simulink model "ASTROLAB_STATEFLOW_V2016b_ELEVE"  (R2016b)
settings: Solver=VariableStepAuto  StartTime=0.0  StopTime=inf  FixedStep=1e-3  MaxStep=0.001  RelTol=1e-3  EnableMultiTasking=on
undefined symbols (not defined in the file): ASTROLAB, CARTER, deg, EMBASE, f, fourche, kg, m, N, r, rad, RootGround, RootPart, s, SIM, STL, tube
libraries: mblibv1 x14, powerlib_meascontrol x4, simulink_extras x4, simulink x1

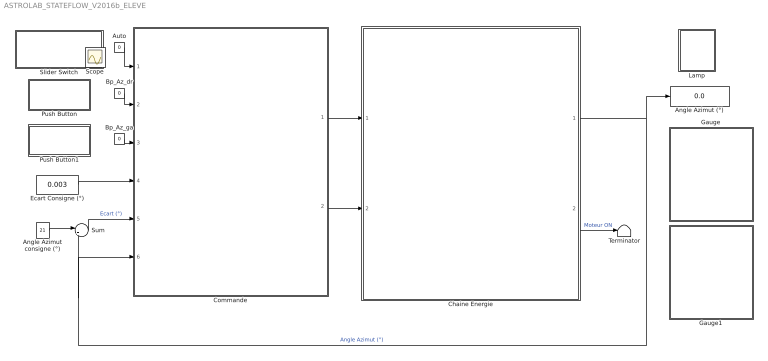
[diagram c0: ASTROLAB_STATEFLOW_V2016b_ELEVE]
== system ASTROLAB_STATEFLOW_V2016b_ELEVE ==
  Angle Azimut consigne (°) : Constant  Value=21
  Angle Azimut (°) : Display
  Auto : Constant  Value=0
  Bp_Az_dr : Constant  Value=0
  Bp_Az_ga : Constant  Value=0
  Chaine Energie : Subsystem
  Commande : Stateflow chart  TreatAsAtomicUnit=on
  Ecart Consigne (°) : Constant  Value=0.003
  Gauge : Subsystem  DialogController=hmiCreateDDGDialog  IsWebBlock=on
  Gauge1 : Subsystem  DialogController=hmiCreateDDGDialog  IsWebBlock=on
  Lamp : Subsystem  DialogController=hmiCreateDDGDialog  IsWebBlock=on
  Push Button : Subsystem  DialogController=hmiCreateDDGDialog  IsWebBlock=on
  Push Button1 : Subsystem  DialogController=hmiCreateDDGDialog  IsWebBlock=on
  Slider Switch : Subsystem  DialogController=hmiCreateDDGDialog  IsWebBlock=on
  Sum : Sum  Inputs=|+-
  Terminator : Terminator
  Scope : Scope
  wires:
  Commande/1(vitesse_azimut) -> Chaine Energie/1(vitesse_azimut)
  Commande/2(sens_azimut) -> Chaine Energie/2(sens_azimut)
  Chaine Energie/1(position_azimut) -> Commande/6(angle_az), Sum/2, Angle Azimut (°)/1  "Angle Azimut (°)"
  Angle Azimut consigne (°)/1 -> Sum/1
  Sum/1 -> Commande/5(e_az)  "Ecart (°)"
  Ecart Consigne (°)/1 -> Commande/4(e_az_cons)
  Auto/1 -> Commande/1(auto)
  Bp_Az_dr/1 -> Commande/2(bp_az_droite)
  Bp_Az_ga/1 -> Commande/3(bp_az_gauche)
  Chaine Energie/2(moteur_on) -> Terminator/1  "Moteur ON"

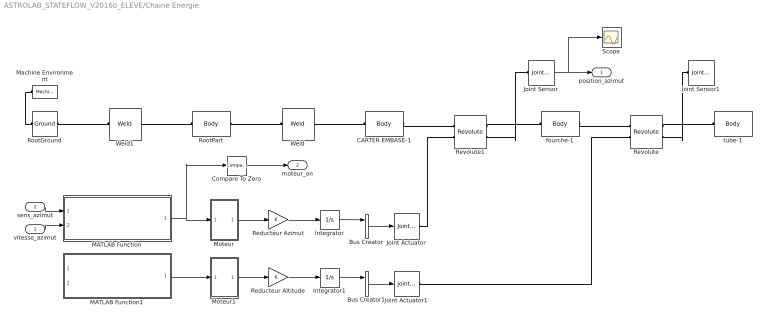
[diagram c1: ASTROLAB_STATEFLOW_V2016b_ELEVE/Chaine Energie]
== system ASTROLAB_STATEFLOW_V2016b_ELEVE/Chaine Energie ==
  vitesse_azimut : Inport
  sens_azimut : Inport  Port=2
  Bus Creator : BusCreator  Inputs=3
  Bus Creator1 : BusCreator  Inputs=3
  CARTER EMBASE-1 : mblibv1/Bodies/Body  LConnTagsString=CS2  RConnTagsString=CS3  UpdateFromCAD=on  PMImportedID=CARTER EMBASE-1  DialogClass=MechanicalBodyBlock  Mass=0.499764  MassUnits=kg  InertiaUnits=kg*m^2  Inertia=[0.0012574,-3.27626e-05,-2.02056e-06;-3.27626e-05,0.00181958,9.31617e-06;-2.02056e-06,9.31617e-06,0.00114593]  Shape=Cylinder  ShapeDims=[1 1]  ShapeUnits=m  ShapeUse=false  Density=1  DensityUnits=kg/m^3  DensityUse=false  GraphicsMode=GFXFILE  GraphicsFileName=STL/ASTROLAB-SIM - CARTER EMBASE-1.STL  BodyColorSelMode=COLORPALETTE  BodyColor=[0.313725;0.313725;0.313725]  AttachedToCS=CS1  CG=Right$CG$[0.000443056 -0.0440147 0.00175883]$WORLD$WORLD$m$[-1 0 0;0 1 0;0 0 -1]$3x3 Transform$rad$WORLD$false$CARTER EMBASE-1::CG(AUTOGEN)  WorkingFrames=Right$CS1$[-0.0385593 -0.0337526 0]$WORLD$WORLD$m$[-1 0 0;0 1 0;0 0 -1]$3x3 Transform$rad$WORLD$false$CARTER EMBASE-1::CS1(AUTOGEN)#Left$CS2$[0.000443056 -0.0440147 0.00175883]$WORLD$WORLD$m$[1 0 0;0 1 0;0 0 1]$3x3 Transform$rad$WORLD$true$ASTROLAB-SIM/RootPart:-:CARTER EMBASE-1::CARTER EMBASE-1(AUTOGEN)#Right$CS3$[0 -0.009 0]$WORLD$WORLD$m$[1 0 0;0 1 0;0 0 1]$3x3 Transform$rad$WORLD$true$CARTER E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  CGPos=[0.000443056 -0.0440147 0.00175883]  CGRot=[-1 0 0;0 1 0;0 0 -1]  CS0Pos=[]  CS0Rot=[]  CS1Pos=[-0.0385593 -0.0337526 0]  CS1Rot=[-1 0 0;0 1 0;0 0 -1]  CS2Pos=[0.000443056 -0.0440147 0.00175883]  CS2Rot=[1 0 0;0 1 0;0 0 1]  CS3Pos=[0 -0.009 0]  CS3Rot=[1 0 0;0 1 0;0 0 1]  CS4Pos=[]  CS4Rot=[]  CS5Pos=[]  CS5Rot=[]  CS6Pos=[]  CS6Rot=[]  CS7Pos=[]  CS7Rot=[]  CS8Pos=[]  CS8Rot=[]  CS9Pos=[]  CS9Rot=[]  CS10Pos=[]  CS10Rot=[]  CS11Pos=[]  CS11Rot=[]  CS12Pos=[]  CS12Rot=[]  CS13Pos=[]  CS13Rot=[]  CS14Pos=[]  CS14Rot=[]  CS15Pos=[]  CS15Rot=[]  CS16Pos=[]  CS16Rot=[]  CS17Pos=[]  CS17Rot=[]  CS18Pos=[]  CS18Rot=[]  CS19Pos=[]  CS19Rot=[]  CS20Pos=[]  CS20Rot=[]
  Compare To Zero : simulink/Logic and Bit Operations/Compare To Zero  relop===  OutDataTypeStr=boolean
  Integrator : Integrator
  Integrator1 : Integrator
  Joint Actuator : mblibv1/Sensors &  Actuators/Joint Actuator  UpdateFromCAD=off  PhysicalDomain=Mechanical  PortType=blob  ActuationStyle=Motion  AngleUnits=rad  ArcVelocityUnits=rad/s  ArcAccelerationUnits=rad/s^2  CoordPositionUnits=m  VelocityUnits=m/s  AccelerationUnits=m/s^2  ForceUnits=N  TorqueUnits=N*m  ActiveIO=on  Width=3  DialogClass=MechanicalActuatorBlock  Primitive=R1  ReferenceFrame=Absolute (World)
  Joint Actuator1 : mblibv1/Sensors &  Actuators/Joint Actuator  UpdateFromCAD=off  PhysicalDomain=Mechanical  PortType=blob  ActuationStyle=Motion  AngleUnits=rad  ArcVelocityUnits=rad/s  ArcAccelerationUnits=rad/s^2  CoordPositionUnits=m  VelocityUnits=m/s  AccelerationUnits=m/s^2  ForceUnits=N  TorqueUnits=N*m  ActiveIO=on  Width=3  DialogClass=MechanicalActuatorBlock  Primitive=R1  ReferenceFrame=Absolute (World)
  Joint Sensor : mblibv1/Sensors &  Actuators/Joint Sensor  UpdateFromCAD=off  PhysicalDomain=Mechanical  PortType=blob  Muxed=off  Pose=off  Angle=on  AngleUnits=deg  ArcVelocity=off  ArcVelocityUnits=deg/s  ArcAcceleration=off  ArcAccelerationUnits=deg/s^2  CoordPosition=on  CoordPositionUnits=mm  Velocity=off  VelocityUnits=m/s  Acceleration=off  AccelerationUnits=m/s^2  Quaternion=on  QuaternionDT=off  QuaternionDDT=off  QuaternionUnits=off  OutputVector=[1]  ActiveIO=on  Width=1  DialogClass=MechanicalSensorBlock  Primitive=R1  Force=off  ForceUnits=N  Torque=off  TorqueUnits=N*m  ReferenceFrame=Absolute (World)  ReactionSensedSide=Base  ReactionReferenceFrame=Absolute (World)  ReactionForce=off  ReactionForceUnits=N  ReactionMoment=off  ReactionMomentUnits=N*m
  Joint Sensor1 : mblibv1/Sensors &  Actuators/Joint Sensor  UpdateFromCAD=off  PhysicalDomain=Mechanical  PortType=blob  Muxed=off  Pose=off  Angle=on  AngleUnits=deg  ArcVelocity=off  ArcVelocityUnits=deg/s  ArcAcceleration=off  ArcAccelerationUnits=deg/s^2  CoordPosition=on  CoordPositionUnits=mm  Velocity=off  VelocityUnits=m/s  Acceleration=off  AccelerationUnits=m/s^2  Quaternion=on  QuaternionDT=off  QuaternionDDT=off  QuaternionUnits=off  OutputVector=[1]  ActiveIO=on  Width=1  DialogClass=MechanicalSensorBlock  Primitive=R1  Force=off  ForceUnits=N  Torque=off  TorqueUnits=N*m  ReferenceFrame=Absolute (World)  ReactionSensedSide=Base  ReactionReferenceFrame=Absolute (World)  ReactionForce=off  ReactionForceUnits=N  ReactionMoment=off  ReactionMomentUnits=N*m
  MATLAB Function : MATLAB Function  TreatAsAtomicUnit=on
  MATLAB Function1 : MATLAB Function  TreatAsAtomicUnit=on
  Machine Environment : mblibv1/Bodies/Machine Environment  PortType=env  PhysicalDomain=Mechanical  DialogTemplateClass=MECH.MachineEnvironment  SyncWhenCopied=off  Gravity=[0 -9.81 0]  GravityUnits=m/s^2  GravityAsSignal=off  Dimensionality=Auto-detect  AnalysisType=Forward dynamics  LinearAssemblyTolerance=1e-3  LinearAssemblyToleranceUnits=m  AngularAssemblyTolerance=1e-3  AngularAssemblyToleranceUnits=rad  ConstraintSolverType=Stabilizing  ConstraintRelTolerance=1e-4  ConstraintAbsTolerance=1e-4  UseRobustSingularityHandling=off  RedundancyAnalysisToleranceType=Automatically select tolerance  RedundancyAnalysisTolerance=1e-14  StatePerturbationType=Fixed  PerturbationSize=1e-5  VisualizeMachine=on  BodyVisualizationType=Use model default body geometries  BodyColorSelMode=Use model default  DefaultBodyColor=[1 0 0]
  Moteur : Subsystem
  Moteur1 : Subsystem
  Reducteur Altitude : Gain
  Reducteur Azimut : Gain
  Revolute : mblibv1/Joints/Revolute  LConnTagsString=__newl0|SA1  RConnTagsString=__newr0|SA1  UpdateFromCAD=on  PMImportedID=fourche-1:-:tube-1  NumSAPorts=2  CutJoint=off  MarkAsCut=off  Primitives=prismatic  PrimitiveProps=R1$World$[0,0,1]$revolute  DialogClass=JointBlock  R1Axis=[0,0,1]
  Revolute1 : mblibv1/Joints/Revolute  LConnTagsString=__newl0|SA1  RConnTagsString=__newr0|SA1  UpdateFromCAD=on  PMImportedID=CARTER EMBASE-1:-:fourche-1  NumSAPorts=2  CutJoint=off  MarkAsCut=off  Primitives=prismatic  PrimitiveProps=R1$World$[0,1,0]$revolute  DialogClass=JointBlock  R1Axis=[0,1,0]
  RootGround : mblibv1/Bodies/Ground  UpdateFromCAD=on  PMImportedID=RootGround  LeftPortType=env  RightPortType=workingframe  PhysicalDomain=Mechanical  DialogClass=GroundBlock  CoordPosition=[-0.0025849,0.0789027,0.00394319]  CoordPositionUnits=m  StateVectorMgrId=-1  MachineId=[0 0]  ShowEnvPort=on  ParameterChecksum=[1257090742, 3741446487, 3378540128, 2534735822]  TopologyChecksum=[924164285, 974059966, 1348323119, 4093688615]
  RootPart : mblibv1/Bodies/Body  LConnTagsString=CS3  RConnTagsString=CS2  UpdateFromCAD=on  PMImportedID=ASTROLAB-SIM/RootPart  DialogClass=MechanicalBodyBlock  Mass=0  MassUnits=kg  InertiaUnits=kg*m^2  Inertia=[0,0,0;0,0,0;0,0,0]  Shape=Cylinder  ShapeDims=[1 1]  ShapeUnits=m  ShapeUse=false  Density=1  DensityUnits=kg/m^3  DensityUse=false  GraphicsMode=MACHINE_DEFAULT  BodyColorSelMode=MACHINE_DEFAULT  BodyColor=[1;0;0]  AttachedToCS=CS1  CG=Right$CG$[-0.0025849 0.0789027 0.00394319]$WORLD$WORLD$m$[1 0 0;0 1 0;0 0 1]$3x3 Transform$rad$WORLD$false$ASTROLAB-SIM/RootPart::CG(AUTOGEN)  WorkingFrames=Right$CS1$[0 0 0]$WORLD$WORLD$m$[1 0 0;0 1 0;0 0 1]$3x3 Transform$rad$WORLD$false$ASTROLAB-SIM/RootPart::CS1(AUTOGEN)#Right$CS2$[0.000443056 -0.0440147 0.00175883]$WORLD$WORLD$m$[1 0 0;0 1 0;0 0 1]$3x3 Transform$rad$WORLD$true$ASTROLAB-SIM/RootPart:-:CARTER EMBASE-1::ASTROLAB-SIM/RootPart(AUTOGEN)#Left$CS3$[-0.0025849 0.0789027 0.00394319]$WORLD$WORLD$m$[1 0 0;0 1 0;0 0 1]$3x3 Transform$rad$WORLD$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  CGPos=[-0.0025849 0.0789027 0.00394319]  CGRot=[1 0 0;0 1 0;0 0 1]  CS0Pos=[]  CS0Rot=[]  CS1Pos=[0 0 0]  CS1Rot=[1 0 0;0 1 0;0 0 1]  CS2Pos=[0.000443056 -0.0440147 0.00175883]  CS2Rot=[1 0 0;0 1 0;0 0 1]  CS3Pos=[-0.0025849 0.0789027 0.00394319]  CS3Rot=[1 0 0;0 1 0;0 0 1]  CS4Pos=[]  CS4Rot=[]  CS5Pos=[]  CS5Rot=[]  CS6Pos=[]  CS6Rot=[]  CS7Pos=[]  CS7Rot=[]  CS8Pos=[]  CS8Rot=[]  CS9Pos=[]  CS9Rot=[]  CS10Pos=[]  CS10Rot=[]  CS11Pos=[]  CS11Rot=[]  CS12Pos=[]  CS12Rot=[]  CS13Pos=[]  CS13Rot=[]  CS14Pos=[]  CS14Rot=[]  CS15Pos=[]  CS15Rot=[]  CS16Pos=[]  CS16Rot=[]  CS17Pos=[]  CS17Rot=[]  CS18Pos=[]  CS18Rot=[]  CS19Pos=[]  CS19Rot=[]  CS20Pos=[]  CS20Rot=[]
  Scope : Scope
  Weld : mblibv1/Joints/Weld  LConnTagsString=__newl0  RConnTagsString=__newr0  UpdateFromCAD=on  PMImportedID=ASTROLAB-SIM/RootPart:-:CARTER EMBASE-1  NumSAPorts=0  CutJoint=off  MarkAsCut=off  Primitives=weld  PrimitiveProps=W$WORLD$[0.57735,0.57735,0.57735]$weld  DialogClass=JointBlock  WAxis=[0.57735,0.57735,0.57735]
  Weld1 : mblibv1/Joints/Weld  LConnTagsString=__newl0  RConnTagsString=__newr0  UpdateFromCAD=on  PMImportedID=ASTROLAB-SIM/RootPart:-:RootGround  NumSAPorts=0  CutJoint=off  MarkAsCut=off  Primitives=weld  PrimitiveProps=W$WORLD$[0.57735,0.57735,0.57735]$weld  DialogClass=JointBlock  WAxis=[0.57735,0.57735,0.57735]
  fourche-1 : mblibv1/Bodies/Body  LConnTagsString=CS3  RConnTagsString=CS2  UpdateFromCAD=on  PMImportedID=fourche-1  DialogClass=MechanicalBodyBlock  Mass=0.514175  MassUnits=kg  InertiaUnits=kg*m^2  Inertia=[0.00244811,5.4534e-05,9.60619e-05;5.4534e-05,0.00280362,-2.46956e-05;9.60619e-05,-2.46956e-05,0.00378344]  Shape=Cylinder  ShapeDims=[1 1]  ShapeUnits=m  ShapeUse=false  Density=1  DensityUnits=kg/m^3  DensityUse=false  GraphicsMode=GFXFILE  GraphicsFileName=STL/ASTROLAB-SIM - fourche-1.STL  BodyColorSelMode=COLORPALETTE  BodyColor=[1;0;0]  AttachedToCS=CS1  CG=Right$CG$[0.000435546 0.0541022 -0.00323293]$WORLD$WORLD$m$[-0.0671397 0 -0.997744;-0.017413 0.999848 0.00117175;0.997592 0.0174524 -0.0671295]$3x3 Transform$rad$WORLD$false$fourche-1::CG(AUTOGEN)  WorkingFrames=Right$CS1$[-0.68803 0.0130791 0.409388]$WORLD$WORLD$m$[-0.0671397 0 -0.997744;-0.017413 0.999848 0.00117175;0.997592 0.0174524 -0.0671295]$3x3 Transform$rad$WORLD$false$fourche-1::CS1(AUTOGEN)#Right$CS2$[6.45282e-07 0.138122 -0.0854162]$WORLD$WORLD$m$[1 0 0;0 1 0;0 0 1]$3x3 Transform$rad$WORLD$true$fourche-1:-:tube-1::fourche-1(AUTOGEN)#Left$CS3$[0 -0.009 0]$WORLD$WORLD$m$[1 0 0;0 1 0;0 0 1]$3x3 T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  CGPos=[0.000435546 0.0541022 -0.00323293]  CGRot=[-0.0671397 0 -0.997744;-0.017413 0.999848 0.00117175;0.997592 0.0174524 -0.0671295]  CS0Pos=[]  CS0Rot=[]  CS1Pos=[-0.68803 0.0130791 0.409388]  CS1Rot=[-0.0671397 0 -0.997744;-0.017413 0.999848 0.00117175;0.997592 0.0174524 -0.0671295]  CS2Pos=[6.45282e-07 0.138122 -0.0854162]  CS2Rot=[1 0 0;0 1 0;0 0 1]  CS3Pos=[0 -0.009 0]  CS3Rot=[1 0 0;0 1 0;0 0 1]  CS4Pos=[]  CS4Rot=[]  CS5Pos=[]  CS5Rot=[]  CS6Pos=[]  CS6Rot=[]  CS7Pos=[]  CS7Rot=[]  CS8Pos=[]  CS8Rot=[]  CS9Pos=[]  CS9Rot=[]  CS10Pos=[]  CS10Rot=[]  CS11Pos=[]  CS11Rot=[]  CS12Pos=[]  CS12Rot=[]  CS13Pos=[]  CS13Rot=[]  CS14Pos=[]  CS14Rot=[]  CS15Pos=[]  CS15Rot=[]  CS16Pos=[]  CS16Rot=[]  CS17Pos=[]  CS17Rot=[]  CS18Pos=[]  CS18Rot=[]  CS19Pos=[]  CS19Rot=[]  CS20Pos=[]  CS20Rot=[]
  tube-1 : mblibv1/Bodies/Body  LConnTagsString=CS2  UpdateFromCAD=on  PMImportedID=tube-1  DialogClass=MechanicalBodyBlock  Mass=1.03705  MassUnits=kg  InertiaUnits=kg*m^2  Inertia=[0.0066886,-0.000601964,0.000159223;-0.000601964,0.00702239,0.000400784;0.000159223,0.000400784,0.00389905]  Shape=Cylinder  ShapeDims=[1 1]  ShapeUnits=m  ShapeUse=false  Density=1  DensityUnits=kg/m^3  DensityUse=false  GraphicsMode=GFXFILE  GraphicsFileName=STL/ASTROLAB-SIM - tube-1.STL  BodyColorSelMode=COLORPALETTE  BodyColor=[0.301961;0.745098;0.933333]  AttachedToCS=CS1  CG=Right$CG$[-0.00554165 0.150434 0.00855382]$WORLD$WORLD$m$[0 0 -1;0 1 0;1 0 0]$3x3 Transform$rad$WORLD$false$tube-1::CG(AUTOGEN)  WorkingFrames=Right$CS1$[6.45282e-07 0.0706217 6.42805e-11]$WORLD$WORLD$m$[0 0 -1;0 1 0;1 0 0]$3x3 Transform$rad$WORLD$false$tube-1::CS1(AUTOGEN)#Left$CS2$[6.45282e-07 0.138122 -0.0854162]$WORLD$WORLD$m$[1 0 0;0 1 0;0 0 1]$3x3 Transform$rad$WORLD$true$fourche-1:-:tube-1::tube-1(AUTOGEN)  CGPos=[-0.00554165 0.150434 0.00855382]  CGRot=[0 0 -1;0 1 0;1 0 0]  CS0Pos=[]  CS0Rot=[]  CS1Pos=[6.45282e-07 0.0706217 6.42805e-11]  CS1Rot=[0 0 -1;0 1 0;1 0 0]  CS2Pos=[6.45282e-07 0.138122 -0.0854162]  CS2Rot=[1 0 0;0 1 0;0 0 1]  CS3Pos=[]  CS3Rot=[]  CS4Pos=[]  CS4Rot=[]  CS5Pos=[]  CS5Rot=[]  CS6Pos=[]  CS6Rot=[]  CS7Pos=[]  CS7Rot=[]  CS8Pos=[]  CS8Rot=[]  CS9Pos=[]  CS9Rot=[]  CS10Pos=[]  CS10Rot=[]  CS11Pos=[]  CS11Rot=[]  CS12Pos=[]  CS12Rot=[]  CS13Pos=[]  CS13Rot=[]  CS14Pos=[]  CS14Rot=[]  CS15Pos=[]  CS15Rot=[]  CS16Pos=[]  CS16Rot=[]  CS17Pos=[]  CS17Rot=[]  CS18Pos=[]  CS18Rot=[]  CS19Pos=[]  CS19Rot=[]  CS20Pos=[]  CS20Rot=[]
  position_azimut : Outport
  moteur_on : Outport  Port=2
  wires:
  vitesse_azimut/1 -> MATLAB Function/2(vitesse_azimut)
  sens_azimut/1 -> MATLAB Function/1(sens_azimut)
  Bus Creator/1 -> Joint Actuator/1
  Joint Sensor/1 -> Scope/1, position_azimut/1
  Bus Creator1/1 -> Joint Actuator1/1
  MATLAB Function1/1(wmot) -> Moteur1/1(In1)
  Integrator/1 -> Bus Creator/1
  Reducteur Azimut/1 -> Integrator/1
  Integrator1/1 -> Bus Creator1/1
  Reducteur Altitude/1 -> Integrator1/1
  Moteur1/1(Out1) -> Reducteur Altitude/1
  MATLAB Function/1(wmot) -> Moteur/1(In1), Compare To Zero/1
  Moteur/1(Out1) -> Reducteur Azimut/1
  Compare To Zero/1 -> moteur_on/1
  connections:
  CARTER EMBASE-1/RConn1 -- Revolute1/LConn1
  Weld1/RConn1 -- RootPart/LConn1
  RootGround/LConn1 -- Machine Environment/RConn1
  RootGround/RConn1 -- Weld1/LConn1
  Revolute/RConn1 -- tube-1/LConn1
  Revolute1/RConn1 -- fourche-1/LConn1
  Weld/RConn1 -- CARTER EMBASE-1/LConn1
  Joint Actuator/RConn1 -- Revolute1/LConn2
  Joint Actuator1/RConn1 -- Revolute/LConn2
  RootPart/RConn1 -- Weld/LConn1
  fourche-1/RConn1 -- Revolute/LConn1
  Joint Sensor/LConn1 -- Revolute1/RConn2
  Joint Sensor1/LConn1 -- Revolute/RConn2

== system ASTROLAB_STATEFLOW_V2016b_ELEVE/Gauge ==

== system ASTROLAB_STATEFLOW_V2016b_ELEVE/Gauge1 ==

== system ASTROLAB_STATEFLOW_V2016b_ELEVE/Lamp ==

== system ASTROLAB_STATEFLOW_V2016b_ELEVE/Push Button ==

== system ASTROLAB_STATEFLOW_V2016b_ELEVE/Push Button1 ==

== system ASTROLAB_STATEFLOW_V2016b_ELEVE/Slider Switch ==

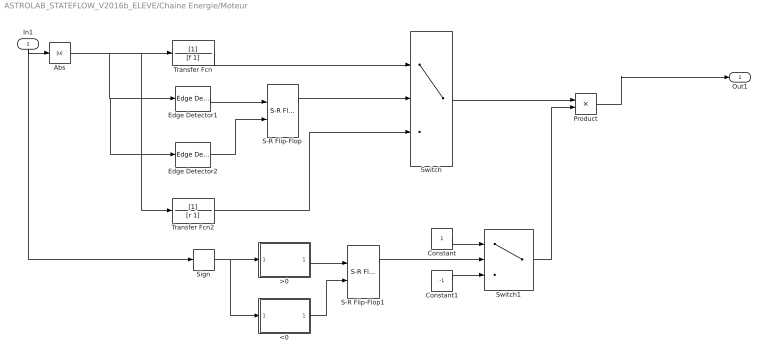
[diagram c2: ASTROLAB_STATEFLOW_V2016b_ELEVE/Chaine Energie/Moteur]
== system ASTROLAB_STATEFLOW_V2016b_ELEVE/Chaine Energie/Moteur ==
  In1 : Inport
  <0 : MATLAB Function  TreatAsAtomicUnit=on
  >0 : MATLAB Function  TreatAsAtomicUnit=on
  Abs : Abs
  Constant : Constant
  Constant1 : Constant  Value=-1
  Edge Detector1 : powerlib_meascontrol/Logic/Edge Detector  model=Falling  ic=0  Ts=0
  Edge Detector2 : powerlib_meascontrol/Logic/Edge Detector  model=Rising  ic=0  Ts=0
  Product : Product
  S-R Flip-Flop : simulink_extras/Flip Flops/S-R Flip-Flop  initial_condition=0
  S-R Flip-Flop1 : simulink_extras/Flip Flops/S-R Flip-Flop  initial_condition=0
  Sign : Signum
  Switch : Switch
  Switch1 : Switch
  Transfer Fcn : TransferFcn  Denominator=[f 1]
  Transfer Fcn2 : TransferFcn  Denominator=[r 1]
  Out1 : Outport
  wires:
  Sign/1 -> <0/1(u), >0/1(u)
  Switch/1 -> Product/1
  Edge Detector2/1 -> S-R Flip-Flop/2
  Transfer Fcn/1 -> Switch/1
  Edge Detector1/1 -> S-R Flip-Flop/1
  S-R Flip-Flop/1 -> Switch/2
  Transfer Fcn2/1 -> Switch/3
  Abs/1 -> Edge Detector2/1, Edge Detector1/1, Transfer Fcn2/1, Transfer Fcn/1
  S-R Flip-Flop1/1 -> Switch1/2
  Constant1/1 -> Switch1/3
  >0/1(y) -> S-R Flip-Flop1/1
  <0/1(y) -> S-R Flip-Flop1/2
  Constant/1 -> Switch1/1
  Switch1/1 -> Product/2
  Product/1 -> Out1/1
  In1/1 -> Abs/1, Sign/1

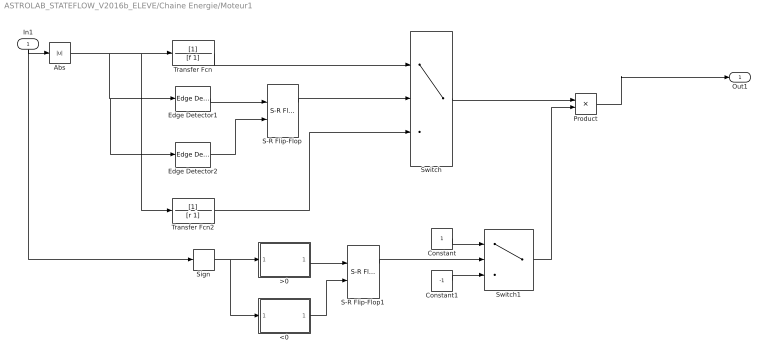
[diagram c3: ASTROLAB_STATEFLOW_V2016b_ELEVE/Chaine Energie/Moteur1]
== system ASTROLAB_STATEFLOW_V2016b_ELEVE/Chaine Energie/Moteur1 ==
  In1 : Inport
  <0 : MATLAB Function  TreatAsAtomicUnit=on
  >0 : MATLAB Function  TreatAsAtomicUnit=on
  Abs : Abs
  Constant : Constant
  Constant1 : Constant  Value=-1
  Edge Detector1 : powerlib_meascontrol/Logic/Edge Detector  model=Falling  ic=0  Ts=0
  Edge Detector2 : powerlib_meascontrol/Logic/Edge Detector  model=Rising  ic=0  Ts=0
  Product : Product
  S-R Flip-Flop : simulink_extras/Flip Flops/S-R Flip-Flop  initial_condition=0
  S-R Flip-Flop1 : simulink_extras/Flip Flops/S-R Flip-Flop  initial_condition=0
  Sign : Signum
  Switch : Switch
  Switch1 : Switch
  Transfer Fcn : TransferFcn  Denominator=[f 1]
  Transfer Fcn2 : TransferFcn  Denominator=[r 1]
  Out1 : Outport
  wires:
  Sign/1 -> <0/1(u), >0/1(u)
  Switch/1 -> Product/1
  Edge Detector2/1 -> S-R Flip-Flop/2
  Transfer Fcn/1 -> Switch/1
  Edge Detector1/1 -> S-R Flip-Flop/1
  S-R Flip-Flop/1 -> Switch/2
  Transfer Fcn2/1 -> Switch/3
  Abs/1 -> Edge Detector2/1, Edge Detector1/1, Transfer Fcn2/1, Transfer Fcn/1
  S-R Flip-Flop1/1 -> Switch1/2
  Constant1/1 -> Switch1/3
  >0/1(y) -> S-R Flip-Flop1/1
  <0/1(y) -> S-R Flip-Flop1/2
  Constant/1 -> Switch1/1
  Switch1/1 -> Product/2
  Product/1 -> Out1/1
  In1/1 -> Abs/1, Sign/1

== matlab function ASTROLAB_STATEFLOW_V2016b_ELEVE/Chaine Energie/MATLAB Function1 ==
function wmot = fcn(sens_altitude,vitesse_altitude)
%#codegen

if sens_altitude == 0
    wmot = 1*vitesse_altitude;
else
    wmot = -1*vitesse_altitude;
end

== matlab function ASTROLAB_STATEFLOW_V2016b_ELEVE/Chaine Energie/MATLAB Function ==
function wmot = fcn(sens_azimut,vitesse_azimut)
%#codegen

if sens_azimut == 0
    wmot = 1*vitesse_azimut; % Remplacer le "1" par la vitesse positive du moteur en rd/s
else
    wmot = -1*vitesse_azimut; % Remplacer le "-1" par la vitesse négative du moteur en rd/s
end

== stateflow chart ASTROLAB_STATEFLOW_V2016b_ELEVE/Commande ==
  state AUTOMATIQUE
    state AUTO_AZIMUT [parallel]
      state AUTO_AZIMUT_STOP
        entry: vitesse_azimut = 0;
      state AUTO_AZIMUT_ATTENTE
        entry: vitesse_azimut = 0;
      state AUTO_AZIMUT_ATTENTE1
        entry: vitesse_azimut = 0;
      state AUTO_AZIMUT_NEGATIF_GV
        entry: vitesse_azimut = 1;
        sens_azimut = 1;
      state AUTO_AZIMUT_POSITIF_GV
        entry: vitesse_azimut = 1;
        sens_azimut = 0;
      (default) -> AUTO_AZIMUT_STOP
      AUTO_AZIMUT_NEGATIF_GV -> AUTO_AZIMUT_STOP
      AUTO_AZIMUT_STOP -> AUTO_AZIMUT_POSITIF_GV : after(40,sec)
      AUTO_AZIMUT_ATTENTE1 -> AUTO_AZIMUT_ATTENTE
      AUTO_AZIMUT_ATTENTE -> AUTO_AZIMUT_NEGATIF_GV
      AUTO_AZIMUT_POSITIF_GV -> AUTO_AZIMUT_ATTENTE1
    state AUTO_ALTITUDE [parallel]
      state Non étudié [group]
  state MANUEL
    state MANUEL_AZIMUT [parallel]
      state MANU_AZIMUT_STOP
        entry: vitesse_azimut = 0;
      state MANU_AZIMUT_NEGATIF_GV
        entry: vitesse_azimut = 1;
        sens_azimut = 1;
      state MANU_AZIMUT_POSITIF_GV
        entry: vitesse_azimut = 1;
        sens_azimut = 0;
      (default) -> MANU_AZIMUT_STOP
      MANU_AZIMUT_POSITIF_GV -> MANU_AZIMUT_STOP
      MANU_AZIMUT_STOP -> MANU_AZIMUT_NEGATIF_GV : after(40,sec)
      MANU_AZIMUT_NEGATIF_GV -> MANU_AZIMUT_POSITIF_GV
    state MANUEL_ALTITUDE [parallel]
      state Non étudié [group]
  MANUEL -> AUTOMATIQUE : [auto == 1]
  (default) -> MANUEL
  AUTOMATIQUE -> MANUEL : [auto == 0]
  data: auto input; bp_az_droite input; bp_az_gauche input; e_az_cons input; vitesse_azimut output; sens_azimut output; e_az input; angle_az input

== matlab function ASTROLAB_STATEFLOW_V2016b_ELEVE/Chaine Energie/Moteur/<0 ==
function y = fcn(u)
%#codegen

if u<0
    y = true;
else
    y = false;
end

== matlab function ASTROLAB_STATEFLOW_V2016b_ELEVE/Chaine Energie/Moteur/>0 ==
function y = fcn(u)
%#codegen

if u>0
    y = true;
else
    y = false;
end

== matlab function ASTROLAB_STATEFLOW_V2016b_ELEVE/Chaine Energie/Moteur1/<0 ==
function y = fcn(u)
%#codegen

if u<0
    y = true;
else
    y = false;
end

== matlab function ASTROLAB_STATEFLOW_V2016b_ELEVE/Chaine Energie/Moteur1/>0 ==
function y = fcn(u)
%#codegen

if u>0
    y = true;
else
    y = false;
end
